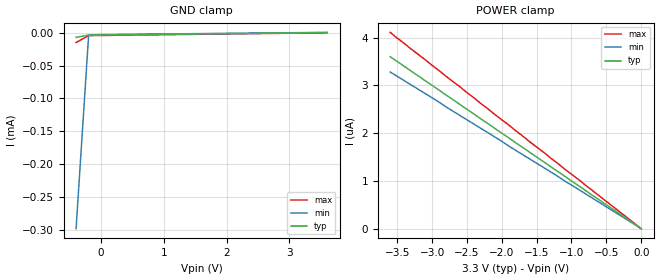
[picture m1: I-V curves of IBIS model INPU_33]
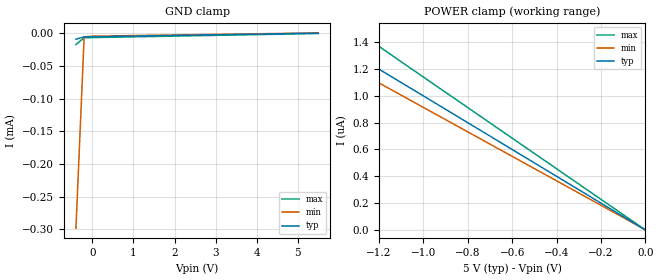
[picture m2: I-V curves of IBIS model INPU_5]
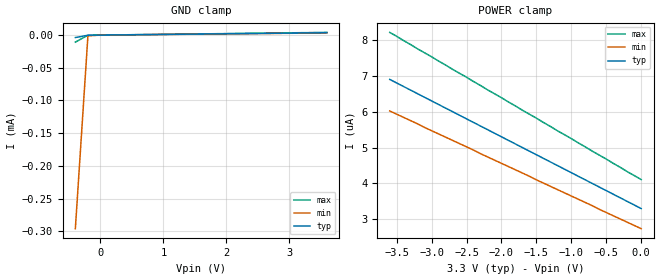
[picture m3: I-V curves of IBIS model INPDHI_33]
|   Texas Instruments Incorporated
|   IBIS Model for ISO723x4x
|   16DW SOIC Package
[IBIS Ver]   4.1
[Comment char]   |_char
[File name]   iso3082.ibs
[File Rev]   1.1
[Date]   October 10, 2018
[Source]
| Texas Instruments Incorporated.
| Analog Design Services, DSS
| 12500 TI Blvd
| Dallas, TX -75243
[Notes]   Revision History:
| Rev 1.1: 10/10/2018
| - Updated models for 3.3V INPU, INPDHI and OUTR
| Rev 1.0: 07/11/2008
| - Initial version of the model
| - Model generated from simulations in TISPICED
[Disclaimer]
| This model is designed as an aid for customers of Texas Instruments.
| TI and its licensors and suppliers make no warranties, either expressed
| or implied, with respect to this  model, including the warranties of
| merchantability or fitness for a particular purpose. The model is
| provided solely on an "as is" basis. The entire risk as to its quality
| and performance is with the customer.
| This model is subject to change without notice. Texas Instruments
| Incorporated is not responsible for updating this model.
[Copyright]
 (C) Copyright 2018 Texas Instruments Incorporated. All rights reserved.
[Component]   ISO3082DW
[Manufacturer]  Texas Instruments Incorporated
[Package]
|   typ   min   max
R_pkg   0.04817   0.03432   0.09530
L_pkg   2.4595nH   1.6904nH   4.7034nH
C_pkg   0.847pF   0.428pF   1.397pF
[Pin]   signal_name   model_name   R_pin   L_pin   C_pin
1   VCC1   POWER   0.03455  3.39778n  0.89677p
2   GND1   GND   0.03432  3.12613n  0.84706p
3   R   OUTR   0.04265  1.85523n  0.57831p
4   REB   INPU   0.03948  1.69049n  0.59300p
5   DE   INPDHI   0.03943  1.70546n  0.55709p
6   D   INPU   0.04257  1.86953n  0.56379p
7   GND1   GND   0.04783  1.99000n  0.60148p
8   GND1   GND   0.03740  4.70338n  1.39696p
9   GND2   GND   0.03763  4.61305n  1.39587p
10   GND2   GND   0.04703  2.01514n  0.58483p
11   NC   NC   0.07132  2.45946n  0.43321p
12   A   DRVR/REC_BI   0.06147  2.13194n  0.42769p
13   B   DRVR/REC_BI   0.07288  2.39260n  0.48001p
14   NC   NC   0.09530  3.03704n  0.47622p
15   GND2   GND   0.04817  4.23145n  0.93567p
16   VCC2   POWER   0.04790  4.51154n  0.99405p
[Diff_pin]   inv_pin   vdiff   tdelay_typ   tdelay_min   tdelay_max
| The 'A' pin is Diff_pin and the 'B' pin is the inv_pin
12   13   0.200   0 0 0
[Model Selector] INPU
INPU_33   REB/D Input model for 3.15V - 3.6V
INPU_5   REB/D Input model for 4.5V - 5.5V
[Model Selector] INPDHI
INPDHI_33   DE Input model for 3.15V - 3.6V
INPDHI_5   DE Input model for 4.5V - 5.5V
[Model Selector] OUTR
OUTR_33   OUTR 3-state output model for 3.0V - 3.6V
OUTR_5   OUTR 3-state output model for 4.5V - 5.5V
| Models and submodels in the file (7): INPU_33 (Input), INPU_5 (Input), INPDHI_33 (Input), INPDHI_5 (Input), OUTR_33 (3-state), OUTR_5 (3-state), DRVR/REC_BI (I/O)
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|   Driver Input / Receiver Enable 3.3V Model
[Model]   INPU_33
Model_type   Input
|Signals   REB,D
Vinl = 0.99
Vinh = 2.31
|   typ   min   max
C_comp   1.3pF   1.1pF   1.5pF
[Model Spec]
Vinl   0.99V   0.945V   1.08V
Vinh   2.31V   2.205V   2.52V
|   typ   min   max
[Temperature Range]   27   -40   125
[Voltage range]   3.3V   3.15V   3.6V
[GND_clamp]
|   Voltage   I(typ)   I(min)   I(max)
-400mV    -7.04uA    -298uA     -14.8uA
-200mV    -3.5uA     -3.91uA    -4.34uA
0V        -3.3uA     -2.74uA    -4.11uA
3.6V      300nA      549nA      14.4pA
[Power_clamp]
| Note that the[POWER_clamp]voltage table is referenced to Vcc
| and is calculated using Vtable=Vcc - Vmeasured.
|   Voltage   I(typ)   I(min)   I(max)
-3.6V     3.6uA      3.28uA     4.11uA
-2.9V     2.9uA      2.65uA     3.31uA
-2.8V     2.8uA      2.55uA     3.19uA
0V        0A         0A         0A
|   Driver Input / Receiver Enable 5V Model
[Model]   INPU_5
Model_type   Input
|Signals   REB,D
Vinh = 2.0
Vinl = 0.8
|   typ   min   max
C_comp   1.3pF   1.1pF   1.5pF
|   typ   min   max
[Temperature Range]   27   -40   85
[Voltage range]   5.0V   4.5V   5.5V
[GND_clamp]
|   Voltage   I(typ)   I(min)   I(max)
-400mV    -8.71uA    -298uA     -16.9uA
-200mV    -5.2uA     -5.27uA    -6.5uA
0V        -5uA       -4.1uA     -6.27uA
5.5V      500nA      913nA      27.5pA
[Power_clamp]
| Note that the[POWER_clamp]voltage table is referenced to Vcc
| and is calculated using Vtable=Vcc - Vmeasured.
|   Voltage   I(typ)   I(min)   I(max)
-5.5V     5.498uA    5.021uA    6.28uA
-1.7V     1.699uA    1.552uA    1.939uA
-1.6V     1.599uA    1.461uA    1.825uA
-1.5V     1.499uA    1.369uA    1.711uA
-1.4V     1.399uA    1.278uA    1.597uA
-1.3V     1.299uA    1.187uA    1.483uA
0V        0A         0A         0A
|   Driver Enable 3.3V
[Model]   INPDHI_33
Model_type   Input
|Signals   DE
Vinh = 2.0
Vinl = 0.8
|   typ   min   max
C_comp   1.3pF   1.1pF   1.5pF
|   typ   min   max
[Temperature Range]   27   -40   85
[Voltage range]   3.3V   3.15V   3.6V
[GND_clamp]
|   Voltage   I(typ)   I(min)   I(max)
-400mV    -3.79uA    -296uA     -10.8uA
-200mV    -202nA     -1.2uA     -230nA
0V        0A         0A         0A
3.6V      3.6uA      3.28uA     4.11uA
[Power_clamp]
| Note that the[POWER_clamp]voltage table is referenced to Vcc
| and is calculated using Vtable=Vcc - Vmeasured.
|   Voltage   I(typ)   I(min)   I(max)
-3.6V     6.9uA      6.02uA     8.21uA
-500mV    3.8uA      3.19uA     4.68uA
-200mV    3.5uA      2.92uA     4.33uA
0V        3.3uA      2.74uA     4.11uA
